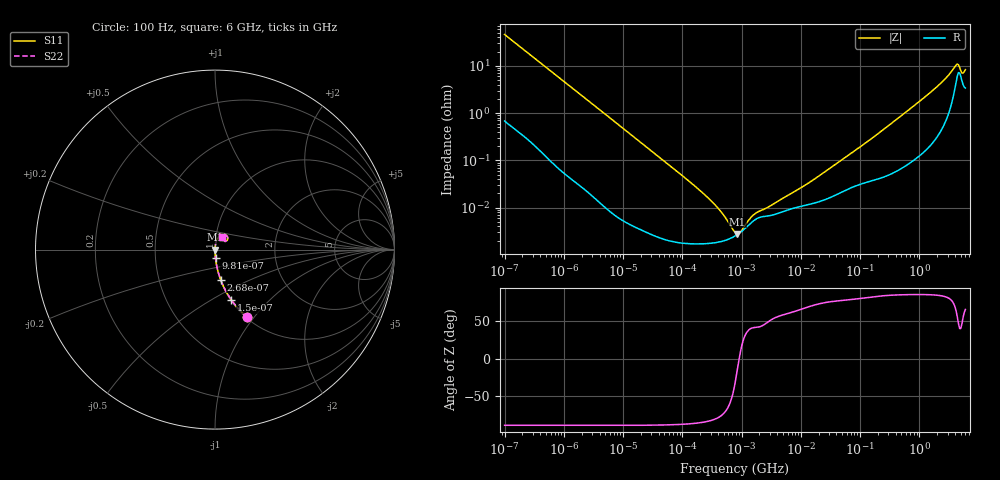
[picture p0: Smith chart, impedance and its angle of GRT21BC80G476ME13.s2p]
!Murata Part Number: GRT21BC80G476ME13
!These Parameters are Measured in Series Mode Connection
!Data Generated on Jun 19, 2026
!  o--ll--o
!Port1  Port2
!  o------o
!Operation Temp=25[degC], DC Bias Voltage=0[V]
!Freq. Start=100[Hz] Stop=6[GHz] 401[Steps]
# Hz S RI R 50
!Freq.(Hz) S11(Real) S11(Imag) S21(Real) S21(Imag) S12(Real) S12(Imag) S22(Real) S22(Imag)
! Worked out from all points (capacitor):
!   401 points, 100 Hz to 6 GHz, reference 50 ohm
!   read as one part in series: C = 34.5 uF near 109 Hz
!   lowest |Z| = 2.79 mohm at 847.2 kHz (marker M1)
!   series resonance near 910.9 kHz, so ESL is about 890 pH
!   S11 on the Smith chart (normalised r, x): 100 Hz: 1.01, -0.92; 150 Hz: 1.01, -0.62; 268 Hz: 1.01, -0.35; 981 Hz: 1.00, -0.10; 6 GHz: 1.07, +0.15
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100  0.1784 -0.3755  0.8216 0.3755  0.8216 0.3755  0.1784 -0.3755
150  0.0904 -0.2795  0.9096 0.2795  0.9096 0.2795  0.0904 -0.2795
268  0.0315 -0.1676  0.9685 0.1676  0.9685 0.1676  0.0315 -0.1676
479  0.0106 -0.0963  0.9894 0.0963  0.9894 0.0963  0.0106 -0.0963
981  0.00283 -0.0477  0.9972 0.0477  0.9972 0.0477  0.00283 -0.0477
2008  0.000821 -0.0235  0.9992 0.0235  0.9992 0.0235  0.000821 -0.0235
40335  2.47e-05 -0.00119  1 0.00119  1 0.00119  2.47e-05 -0.00119
176758  1.72e-05 -0.000262  1 0.000262  1 0.000262  1.72e-05 -0.000262
378399  1.84e-05 -0.000104  1 0.000104  1 0.000104  1.84e-05 -0.000104
432798  1.9e-05 -8.51e-05  1 8.51e-05  1 8.51e-05  1.9e-05 -8.51e-05
774597  2.51e-05 -1.65e-05  1 1.65e-05  1 1.65e-05  2.51e-05 -1.65e-05
847162  2.7e-05 -7.2e-06  1 7.2e-06  1 7.2e-06  2.7e-05 -7.2e-06
2837864  6.69e-05 7.87e-05  0.9999 -7.87e-05  0.9999 -7.87e-05  6.69e-05 7.87e-05
1.555665e7  0.000122 0.000354  0.9999 -0.000354  0.9999 -0.000354  0.000122 0.000354
1.066761e8  0.000324 0.00201  0.9997 -0.00201  0.9997 -0.00201  0.000324 0.00201
3.124326e8  0.000527 0.00559  0.9995 -0.00559  0.9995 -0.00559  0.000527 0.00559
1.873145e9  0.00391 0.0335  0.9961 -0.0335  0.9961 -0.0335  0.00391 0.0335
2.802721e9  0.00968 0.0535  0.9903 -0.0535  0.9903 -0.0535  0.00968 0.0535
4.009986e9  0.0405 0.0842  0.9595 -0.0842  0.9595 -0.0842  0.0405 0.0842
4.385646e9  0.0641 0.0794  0.9359 -0.0794  0.9359 -0.0794  0.0641 0.0794
5.245841e9  0.0483 0.0469  0.9517 -0.0469  0.9517 -0.0469  0.0483 0.0469
6e9  0.0379 0.0706  0.9621 -0.0706  0.9621 -0.0706  0.0379 0.0706
